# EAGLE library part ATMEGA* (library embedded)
MICROCONTROLLER 64/128/256 Kbytes FLASH 4 Kbytes EEPROM 8 Kbytes SRAM 86 General Purpose I/O pins 12-channels16-bit PWM 4 x Serial USARTs 16-channels 10-bit A/D
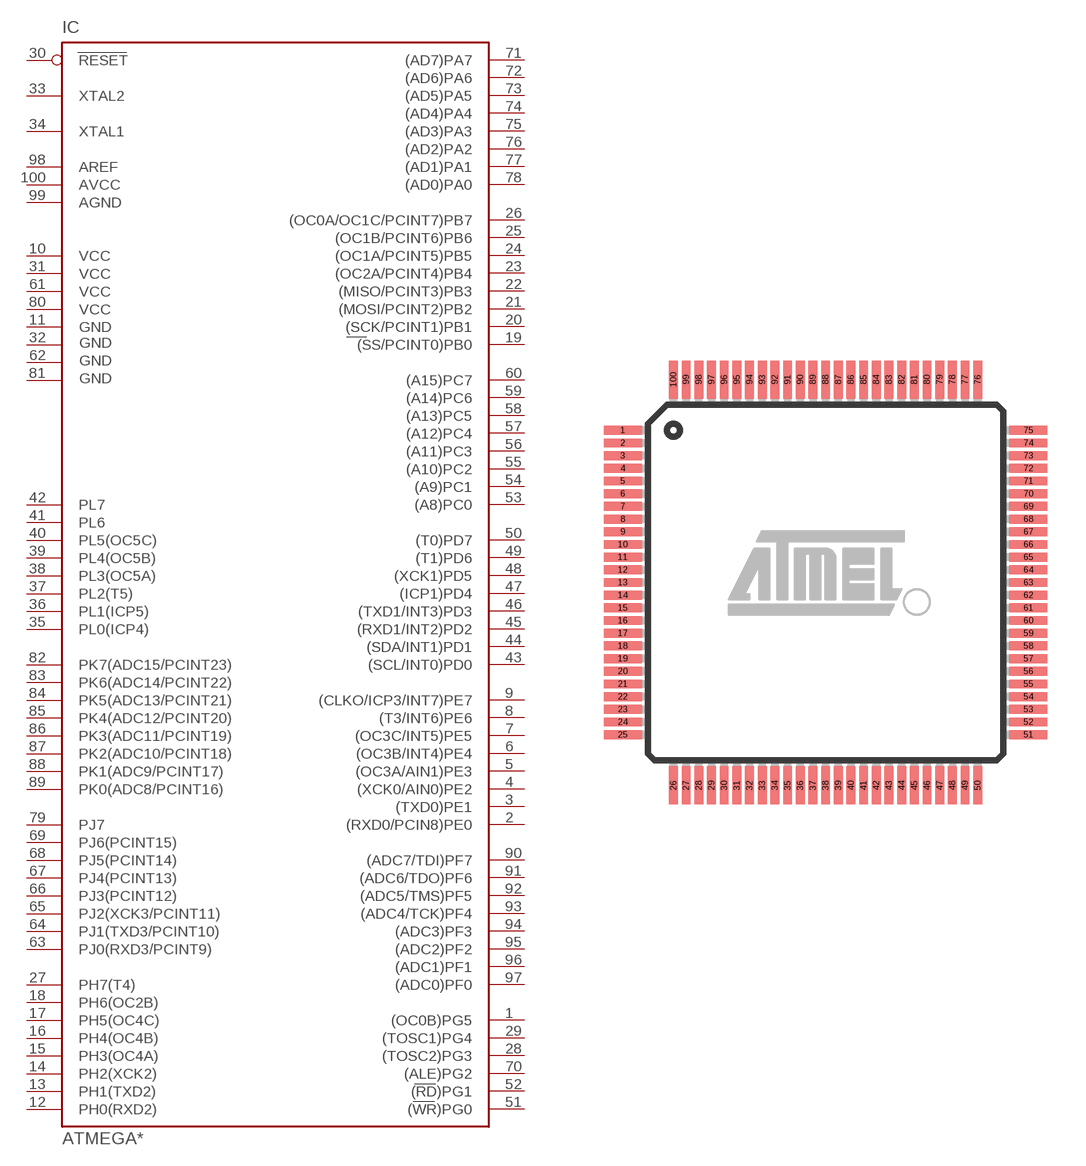
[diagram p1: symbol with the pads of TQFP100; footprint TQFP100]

Designator prefix IC

## ATMEGA1280-16AI, ATMEGA1280V-8AI, ATMEGA2560-16AI, ATMEGA2560V-8AI, ATMEGA640-16AI, ATMEGA640V-8AI  [TQFP100]
1  (OC0B)PG5
2  (RXD0/PCIN8)PE0
3  (TXD0)PE1
4  (XCK0/AIN0)PE2
5  (OC3A/AIN1)PE3
6  (OC3B/INT4)PE4
7  (OC3C/INT5)PE5
8  (T3/INT6)PE6
9  (CLKO/ICP3/INT7)PE7
10  VCC  pwr
11  GND  pwr
12  PH0(RXD2)
13  PH1(TXD2)
14  PH2(XCK2)
15  PH3(OC4A)
16  PH4(OC4B)
17  PH5(OC4C)
18  PH6(OC2B)
19  (SS/PCINT0)PB0
20  (SCK/PCINT1)PB1
21  (MOSI/PCINT2)PB2
22  (MISO/PCINT3)PB3
23  (OC2A/PCINT4)PB4
24  (OC1A/PCINT5)PB5
25  (OC1B/PCINT6)PB6
26  (OC0A/OC1C/PCINT7)PB7
27  PH7(T4)
28  (TOSC2)PG3
29  (TOSC1)PG4
30  RESET  in
31  VCC1  pwr
32  GND1  pwr
33  XTAL2  out
34  XTAL1  in
35  PL0(ICP4)
36  PL1(ICP5)
37  PL2(T5)
38  PL3(OC5A)
39  PL4(OC5B)
40  PL5(OC5C)
41  PL6
42  PL7
43  (SCL/INT0)PD0
44  (SDA/INT1)PD1
45  (RXD1/INT2)PD2
46  (TXD1/INT3)PD3
47  (ICP1)PD4
48  (XCK1)PD5
49  (T1)PD6
50  (T0)PD7
51  (WR)PG0
52  (RD)PG1
53  (A8)PC0
54  (A9)PC1
55  (A10)PC2
56  (A11)PC3
57  (A12)PC4
58  (A13)PC5
59  (A14)PC6
60  (A15)PC7
61  VCC2  pwr
62  GND2  pwr
63  PJ0(RXD3/PCINT9)
64  PJ1(TXD3/PCINT10)
65  PJ2(XCK3/PCINT11)
66  PJ3(PCINT12)
67  PJ4(PCINT13)
68  PJ5(PCINT14)
69  PJ6(PCINT15)
70  (ALE)PG2
71  (AD7)PA7
72  (AD6)PA6
73  (AD5)PA5
74  (AD4)PA4
75  (AD3)PA3
76  (AD2)PA2
77  (AD1)PA1
78  (AD0)PA0
79  PJ7
80  VCC3  pwr
81  GND3  pwr
82  PK7(ADC15/PCINT23)
83  PK6(ADC14/PCINT22)
84  PK5(ADC13/PCINT21)
85  PK4(ADC12/PCINT20)
86  PK3(ADC11/PCINT19)
87  PK2(ADC10/PCINT18)
88  PK1(ADC9/PCINT17)
89  PK0(ADC8/PCINT16)
90  (ADC7/TDI)PF7
91  (ADC6/TDO)PF6
92  (ADC5/TMS)PF5
93  (ADC4/TCK)PF4
94  (ADC3)PF3
95  (ADC2)PF2
96  (ADC1)PF1
97  (ADC0)PF0
98  AREF
99  AGND  pwr
100  AVCC  pwr

## ATMEGA1280-16AU, ATMEGA1280V-8AU, ATMEGA2560-16AU (DATASHEET: http://ww1.microchip.com/downloads/en/DeviceDoc/Atmel-2549-8-bit-AVR-Microcontroller-ATmega640-1280-1281-2560-2561_datasheet.pdf; DESCR: 8-bit Microcontrollers - MCU 256kB Flash 4kB EEPROM 86 I/O Pins; FARNELL_NO: 1288330; MF: Atmel; MF_PN: ATMEGA2560-16AU; MOUSER_NO: 556-ATMEGA2560-16AU; PACKAGE: TQFP-100; PURCHASE: https://de.farnell.com/atmel/atmega2560-16au/8bit-mcu-256k-flash-5v-smd-2560/dp/1288330; UNIT_PRICE: 10.13), ATMEGA2560V-8AU, ATMEGA640-16AU, ATMEGA640V-8AU  [TQFP100]
Pads as for TQFP100

## Footprint TQFP100 (pad centres in mm)
100-lead Thin Quad Flat Pack Package Outline
smd 1.5 x 0.35: 1 -8,6; 2 -8,5.5; 3 -8,5; 4 -8,4.5; 5 -8,4; 6 -8,3.5; 7 -8,3; 8 -8,2.5; 9 -8,2; 10 -8,1.5; 11 -8,1; 12 -8,0.5; 13 -8,0; 14 -8,-0.5; 15 -8,-1; 16 -8,-1.5; 17 -8,-2; 18 -8,-2.5; 19 -8,-3; 20 -8,-3.5; 21 -8,-4; 22 -8,-4.5; 23 -8,-5; 24 -8,-5.5; 25 -8,-6; 51 8,-6; 52 8,-5.5; 53 8,-5; 54 8,-4.5; 55 8,-4; 56 8,-3.5; 57 8,-3; 58 8,-2.5; 59 8,-2; 60 8,-1.5; 61 8,-1; 62 8,-0.5; 63 8,0; 64 8,0.5; 65 8,1; 66 8,1.5; 67 8,2; 68 8,2.5; 69 8,3; 70 8,3.5; 71 8,4; 72 8,4.5; 73 8,5; 74 8,5.5; 75 8,6
smd 0.35 x 1.5: 26 -6,-8; 27 -5.5,-8; 28 -5,-8; 29 -4.5,-8; 30 -4,-8; 31 -3.5,-8; 32 -3,-8; 33 -2.5,-8; 34 -2,-8; 35 -1.5,-8; 36 -1,-8; 37 -0.5,-8; 38 0,-8; 39 0.5,-8; 40 1,-8; 41 1.5,-8; 42 2,-8; 43 2.5,-8; 44 3,-8; 45 3.5,-8; 46 4,-8; 47 4.5,-8; 48 5,-8; 49 5.5,-8; 50 6,-8; 76 6,8; 77 5.5,8; 78 5,8; 79 4.5,8; 80 4,8; 81 3.5,8; 82 3,8; 83 2.5,8; 84 2,8; 85 1.5,8; 86 1,8; 87 0.5,8; 88 0,8; 89 -0.5,8; 90 -1,8; 91 -1.5,8; 92 -2,8; 93 -2.5,8; 94 -3,8; 95 -3.5,8; 96 -4,8; 97 -4.5,8; 98 -5,8; 99 -5.5,8; 100 -6,8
